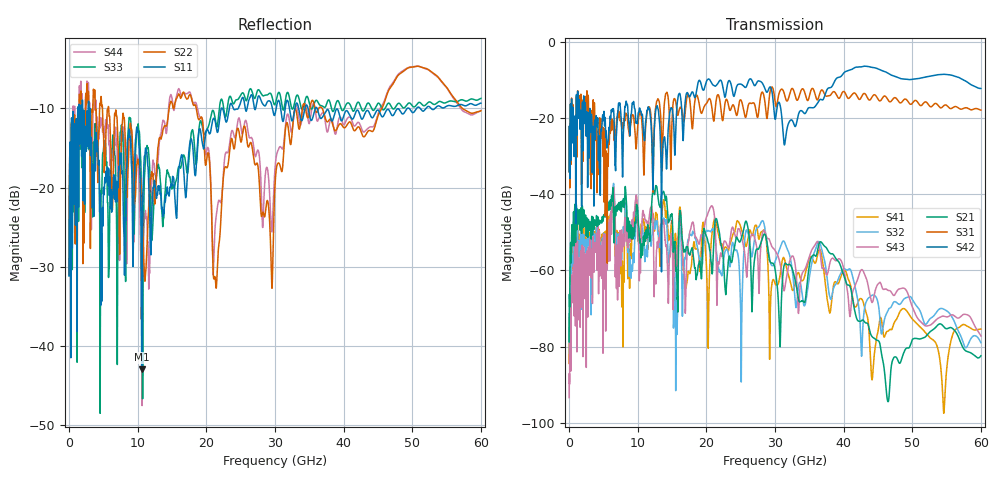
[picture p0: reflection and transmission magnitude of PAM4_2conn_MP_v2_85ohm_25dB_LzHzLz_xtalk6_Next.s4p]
! Info: Touchstone file created by Circ.  Input file=FAB50GbE_2conn_Midplane_Examax_Topo2_v2_85ohm_25dB_LzHzLz.circ
# Hz S RI R 50
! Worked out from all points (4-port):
!   6000 points, 10 MHz to 60 GHz, reference 50 ohm
!   strongest paths, dB at 10 MHz, 15.01 GHz, 30.01 GHz, 45.01 GHz, 60 GHz:
!     S42: -34.0, -17.4, -20.2, -7.0, -12.1
!     S31: -34.0, -20.4, -15.4, -14.9, -17.8
!     S21: -78.8, -45.4, -59.6, -78.4, -82.4
!     S43: -93.4, -51.9, -54.7, -63.6, -77.2
!     S32: -78.6, -50.8, -57.7, -68.5, -79.0
!     S41: -84.4, -47.2, -63.5, -76.1, -75.4
!   lowest |S11| = -43.0 dB at 10.58 GHz (marker M1), VSWR 1.01, Z = 50.3 - j0.635 ohm
!   |S11| at or under -10 dB: start of sweep to 1.267 GHz; 3.036 GHz to 22.18 GHz (19.15 GHz wide, 152 % of centre); 36.15 GHz to 49.26 GHz (13.11 GHz wide, 30.7 % of centre)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
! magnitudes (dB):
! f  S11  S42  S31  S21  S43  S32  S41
! 10 MHz  -31.2  -34.0  -34.0  -78.8  -93.4  -78.6  -84.4
! 1.08 GHz  -11.5  -13.7  -14.2  -43.1  -55.6  -50.7  -49.4
! 10.58 GHz  -43.0  -19.2  -20.3  -53.0  -49.9  -49.4  -47.9
! 15.96 GHz  -18.0  -13.7  -18.5  -52.4  -50.6  -52.9  -48.5
! 20.27 GHz  -12.8  -9.6  -15.2  -52.7  -44.7  -49.5  -80.4
! 21.29 GHz  -11.6  -11.5  -17.6  -47.0  -48.6  -51.7  -46.3
! 60 GHz  -9.3  -12.1  -17.8  -82.4  -77.2  -79.0  -75.4
